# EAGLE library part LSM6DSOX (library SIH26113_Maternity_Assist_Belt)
ST LSM6DSOXTR 6-axis IMU (3-axis accel + 3-axis gyro), LGA-14L. Pin map from LSM6DSOX DS12814 Rev.4 Table 1.
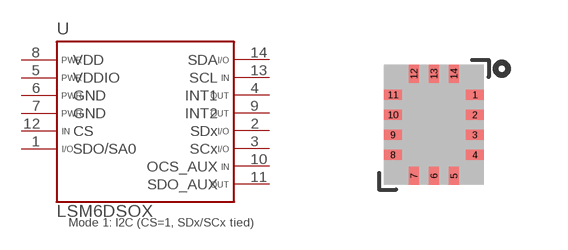
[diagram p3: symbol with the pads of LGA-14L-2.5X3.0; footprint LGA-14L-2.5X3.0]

Designator prefix U

## LSM6DSOX  [LGA-14L-2.5X3.0]
1  SDO/SA0
2  SDx
3  SCx
4  INT1  out
5  VDDIO  pwr
6  GND  pwr
7  GND  pwr
8  VDD  pwr
9  INT2  out
10  OCS_AUX  in
11  SDO_AUX  out
12  CS  in
13  SCL  in
14  SDA

## Footprint LGA-14L-2.5X3.0 (pad centres in mm)
ST LGA-14L 2.5x3.0x0.86 mm. Body/pad geometry from LSM6DSOX DS12814 Rev.4 Fig.28 (14 pads 0.475x0.25 mm, 0.5 mm pitch, 1.5/1.0 mm row spans). Lands enlarged to 0.50x0.28 mm per IPC-7351B Nominal.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
smd 0.45 x 0.25: 1 1.025,0.75; 2 1.025,0.25; 3 1.025,-0.25; 4 1.025,-0.75; 8 -1.025,-0.75; 9 -1.025,-0.25; 10 -1.025,0.25; 11 -1.025,0.75
smd 0.25 x 0.45: 5 0.5,-1.275; 6 0,-1.275; 7 -0.5,-1.275; 12 -0.5,1.275; 13 0,1.275; 14 0.5,1.275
